| IBIS file was generated by Viper version: 2024.10.21
[IBIS Ver]   4.2
[Comment Char]   |_char
[File Name]   mcxl20_184mapbga_9x9_l25x.ibs
[File Rev]   1.0
[Date]   Thu Oct 24 12:27:40 2024
[Source]   NXP Viper 2024.10.21
[Notes]
[Disclaimer] IMPORTANT NOTICE
  This information is provided on an AS IS basis and without warranty.
  IN NO EVENT SHALL NXP BE LIABLE FOR INCIDENTAL OR CONSEQUENTIAL
  DAMAGES ARISING FROM USE OF THIS INFORMATION. THIS DISCLAIMER OF
  WARRANTY EXTENDS TO THE USER OF THE INFORMATION, AND TO THEIR CUSTOMERS
  OR USERS OF PRODUCTS  AND IS IN LIEU OF ALL WARRANTIES WHETHER EXPRESS,
  IMPLIED, OR STATUTORY, INCLUDING IMPLIED WARRANTIES OF MERCHANTABILITY
  OR FITNESS FOR PARTICULAR PURPOSE.
  NXP does not represent or warrant that the information furnished
  hereunder is free of infringement of any third party patents,
  copyrights, trade secrets, or other intellectual property rights.
  NXP does not represent or warrant that the information is free of
  defect, or that it meets any particular standard, requirements or need
  of the user of the infomation or their customers.
  NXP reserves the right to change the information in this file
  without notice.
   http://www.nxp.com
[Copyright]   (C) Copyright NXP 2004 - 2024, All Rights Reserved.
|   MCXL20_184MAPBGA_9x9_L25x
[Component]   MCXL20_184MAPBGA_9x9_L25x
[Manufacturer]   NXP
[Package]
| variable   typ   min   max
R_pkg   0.15423   0.065679   0.22133
L_pkg   2.171e-09   9.268e-10   3.289e-09
C_pkg   5.439e-13   4.158e-13   9.414e-13
[Pin] signal_name   model_name   R_pin   L_pin   C_pin
A1   P1_13   a_ip_io_3v_3p3v   0.17035   3.190e-09 4.598e-13
A2   P1_12   a_ip_io_3v_3p3v   0.17872   3.289e-09 4.578e-13
A4   P1_8   a_ip_io_3v_3p3v   0.1711   2.737e-09 4.589e-13
A6   P1_5   a_ip_io_3v_3p3v   0.147   2.098e-09 5.293e-13
A8   P1_1   a_ip_io_3v_3p3v   0.16054   2.231e-09 5.120e-13
A10   P0_17   a_ip_io_3v_3p3v   0.17426   2.236e-09 5.511e-13
A12   P0_13   a_ip_io_3v_3p3v   0.18672   2.413e-09 5.370e-13
A14   P0_11   a_ip_io_3v_3p3v   0.18543   2.630e-09 6.485e-13
A16   P0_7   a_ip_io_3v_3p3v   0.20755   2.993e-09 6.875e-13
A17   P0_6   a_ip_io_3v_3p3v   0.20761   2.937e-09 6.404e-13
B1   P1_14   a_ip_io_3v_3p3v   0.19608   3.271e-09 4.663e-13
B2   P1_11   a_ip_io_3v_3p3v   0.15597   2.797e-09 4.421e-13
B3   P1_10   a_ip_io_3v_3p3v   0.15222   2.391e-09 4.507e-13
B4   P1_9   a_ip_io_3v_3p3v   0.1519   2.545e-09 4.674e-13
B6   P1_4   a_ip_io_3v_3p3v   0.13797   1.822e-09 5.117e-13
B7   P1_3   a_ip_io_3v_3p3v   0.13944   1.902e-09 5.174e-13
B8   P1_2   a_ip_io_3v_3p3v   0.15785   2.105e-09 5.004e-13
B10   P0_16   a_ip_io_3v_3p3v   0.1414   1.899e-09 5.304e-13
B11   P0_15   a_ip_io_3v_3p3v   0.15716   2.043e-09 5.124e-13
B12   P0_14   a_ip_io_3v_3p3v   0.14993   2.047e-09 5.325e-13
B14   P0_10   a_ip_io_3v_3p3v   0.19084   2.566e-09 6.231e-13
B15   P0_9   a_ip_io_3v_3p3v   0.17659   2.485e-09 6.402e-13
B16   P0_8   a_ip_io_3v_3p3v   0.20374   2.822e-09 6.714e-13
B17   P0_5   a_ip_io_3v_3p3v   0.1786   2.546e-09 6.374e-13
C3   P1_15   a_ip_io_3v_3p3v   0.1334   2.475e-09 4.406e-13
C4   P1_7   a_ip_io_3v_3p3v   0.13148   2.019e-09 4.158e-13
C5   P1_6   a_ip_io_3v_3p3v   0.12228   1.611e-09 4.344e-13
C6   VSS   GND   NA   NA   NA
C8   P1_0   a_ip_io_3v_3p3v   0.13521   1.593e-09 5.029e-13
C9   VSS   GND   NA   NA   NA
C10   VDD   POWER   NA   NA   NA
C12   VDD_ANA_LPADC   POWER   NA   NA   NA
C13   VSS   GND   NA   NA   NA
C14   P0_12   a_ip_io_3v_3p3v   0.17111   2.212e-09 5.976e-13
C15   RESET_B   NC   0.15386   2.028e-09 5.733e-13
D1   P1_18   a_ip_io_3v_3p3v   0.22133   2.968e-09 4.908e-13
D2   P1_17   a_ip_io_3v_3p3v   0.1529   2.346e-09 4.588e-13
D3   P1_16   a_ip_io_3v_3p3v   0.14234   2.267e-09 4.313e-13
D4   VDD   POWER   NA   NA   NA
D6   VSS   GND   NA   NA   NA
D7   NC   NC   NA   NA   NA
D9   VDD   POWER   NA   NA   NA
D11   VDD_ANA_LPADC   POWER   NA   NA   NA
D12   NC   NC   NA   NA   NA
D14   VSS   GND   NA   NA   NA
D15   VSS   GND   NA   NA   NA
D16   RTC_XO   NC   0.18344   2.356e-09 5.402e-13
D17   RTC_XI   NC   0.18384   2.393e-09 5.692e-13
E4   VSS   GND   NA   NA   NA
E5   VDD   POWER   NA   NA   NA
E7   NC   NC   NA   NA   NA
E8   NC   NC   NA   NA   NA
E10   VSS   GND   NA   NA   NA
E11   NC   NC   NA   NA   NA
E13   NC   NC   NA   NA   NA
E14   POR_EXT_B   NC   0.10978   1.409e-09 5.465e-13
F1   P1_20   a_ip_io_3v_3p3v   0.18086   2.509e-09 5.643e-13
F2   P1_21   a_ip_io_3v_3p3v   0.14346   2.018e-09 5.346e-13
F3   P1_19   a_ip_io_3v_3p3v   0.12864   1.985e-09 5.199e-13
F4   VSS   GND   NA   NA   NA
F6   NC   NC   NA   NA   NA
F8   NC   NC   NA   NA   NA
F10   NC   NC   NA   NA   NA
F12   NC   NC   NA   NA   NA
F14   ATESTMODE   NC   0.11304   1.279e-09 5.081e-13
F15   P0_4   a_ip_io_3v_3p3v   0.14348   1.835e-09 5.189e-13
F16   P0_2   a_ip_io_3v_3p3v   0.13975   1.819e-09 4.673e-13
F17   P0_3   a_ip_io_3v_3p3v   0.14535   2.001e-09 5.299e-13
G2   P1_22   a_ip_io_3v_3p3v   0.13527   1.813e-09 5.193e-13
G4   NC   NC   NA   NA   NA
G5   NC   NC   NA   NA   NA
G7   NC   NC   NA   NA   NA
G11   NC   NC   NA   NA   NA
G13   VSS   GND   NA   NA   NA
G14   NC   NC   NA   NA   NA
G16   P0_1   a_ip_io_3v_3p3v   0.142   1.967e-09 5.272e-13
H1   P2_1   a_ip_io_3v_3p3v   0.15528   2.115e-09 5.171e-13
H2   P2_0   a_ip_io_3v_3p3v   0.14258   1.997e-09 5.196e-13
H3   P2_2   a_ip_io_3v_3p3v   0.11824   1.636e-09 5.203e-13
H5   VSS   GND   NA   NA   NA
H6   NC   NC   NA   NA   NA
H8   VSS   GND   NA   NA   NA
H9   VSS   GND   NA   NA   NA
H10   VSS   GND   NA   NA   NA
H12   NC   NC   NA   NA   NA
H13   VDD_CORE_AON   POWER   NA   NA   NA
H15   VOUT_RTC   POWER   0.066449  9.268e-10 5.631e-13
H16   P0_0   a_ip_io_3v_3p3v   0.11817   1.686e-09 5.084e-13
H17   VOUT_SNS   POWER   0.096977  1.574e-09 6.065e-13
J3   P2_3   a_ip_io_3v_3p3v   0.1384   1.795e-09 4.931e-13
J4   VSS   GND   NA   NA   NA
J8   VSS   GND   NA   NA   NA
J10   VSS   GND   NA   NA   NA
J14   VSS   GND   NA   NA   NA
J15   VDD_CORE_AON   POWER   NA   NA   NA
K1   P2_5   a_ip_io_3v_3p3v   0.16205   2.076e-09 4.792e-13
K2   VDD   POWER   NA   NA   NA
K3   P2_4   a_ip_io_3v_3p3v   0.11659   1.536e-09 4.922e-13
K5   NC   NC   NA   NA   NA
K6   NC   NC   NA   NA   NA
K8   VSS   GND   NA   NA   NA
K9   VSS   GND   NA   NA   NA
K10   VSS   GND   NA   NA   NA
K12   NC   NC   NA   NA   NA
K13   VDD   POWER   NA   NA   NA
K15   VSS   GND   NA   NA   NA
K16   DCDC_BUCK_LX_AON   NC   0.06933   1.352e-09 7.820e-13
K17   VSS_DCDC_BUCK   GND   NA   NA   NA
L2   VSS   GND   NA   NA   NA
L4   VDD   POWER   NA   NA   NA
L5   VSS   GND   NA   NA   NA
L7   VDD_CORE_FIXED   POWER   NA   NA   NA
L11   NC   NC   NA   NA   NA
L13   NC   NC   NA   NA   NA
L14   VDD_BAT   POWER   NA   NA   NA
L16   VDD_BAT   POWER   NA   NA   NA
M1   P2_7   a_ip_io_3v_3p3v   0.14505   2.265e-09 5.355e-13
M2   P2_6   a_ip_io_3v_3p3v   0.15877   2.334e-09 5.294e-13
M3   VSS   GND   NA   NA   NA
M4   VSS   GND   NA   NA   NA
M6   NC   NC   NA   NA   NA
M8   NC   NC   NA   NA   NA
M10   VDD   POWER   NA   NA   NA
M12   NC   NC   NA   NA   NA
M14   VSS   GND   NA   NA   NA
M15   VSS   GND   NA   NA   NA
M16   DCDC_BUCK_LX_FIXED   NC   0.065679  1.036e-09 9.414e-13
M17   VSS_DCDC_BUCK   GND   NA   NA   NA
N4   P2_8   a_ip_io_3v_3p3v   0.14427   2.164e-09 5.628e-13
N5   VSS   GND   NA   NA   NA
N7   NC   NC   NA   NA   NA
N8   NC   NC   NA   NA   NA
N10   VSS   GND   NA   NA   NA
N11   NC   NC   NA   NA   NA
N13   VSS   GND   NA   NA   NA
N14   VDD   POWER   NA   NA   NA
P1   P2_9   a_ip_io_3v_3p3v   0.15939   2.256e-09 5.746e-13
P2   P2_10   a_ip_io_3v_3p3v   0.15955   2.136e-09 5.217e-13
P3   P2_11   a_ip_io_3v_3p3v   0.12991   1.777e-09 4.989e-13
P4   VDD   POWER   NA   NA   NA
P6   VSS   GND   NA   NA   NA
P7   NC   NC   NA   NA   NA
P9   VDD_ANA   POWER   NA   NA   NA
P11   VSS   GND   NA   NA   NA
P12   NC   NC   NA   NA   NA
P14   P3_15   a_ip_io_3v_3p3v   0.1417   1.812e-09 5.514e-13
P15   P3_12   a_ip_io_3v_3p3v   0.13965   1.919e-09 5.073e-13
P16   P3_13   a_ip_io_3v_3p3v   0.15542   2.050e-09 5.457e-13
P17   P3_14   a_ip_io_3v_3p3v   0.16043   2.203e-09 5.670e-13
R3   P2_12   a_ip_io_3v_3p3v   0.17829   2.525e-09 5.424e-13
R4   VDD   POWER   NA   NA   NA
R5   VSS   GND   NA   NA   NA
R6   VDD_CORE_FIXED   POWER   NA   NA   NA
R8   P2_25   a_ip_io_3v_3p3v   0.13425   1.649e-09 5.066e-13
R9   VDD_ANA   POWER   NA   NA   NA
R10   VREFH   NC   0.1028   1.380e-09 5.570e-13
R12   P3_1   a_ip_io_3v_3p3v   0.135   1.746e-09 5.163e-13
R13   P3_2   a_ip_io_3v_3p3v   0.12852   1.785e-09 5.125e-13
R14   P3_3   a_ip_io_3v_3p3v   0.16046   2.284e-09 4.923e-13
R15   P3_11   a_ip_io_3v_3p3v   0.12561   1.727e-09 4.876e-13
T1   P2_13   a_ip_io_3v_3p3v   0.16973   2.448e-09 5.851e-13
T2   P2_16   a_ip_io_3v_3p3v   0.15512   2.189e-09 5.473e-13
T3   P2_17   a_ip_io_3v_3p3v   0.16722   2.231e-09 5.754e-13
T4   P2_18   a_ip_io_3v_3p3v   0.16507   2.238e-09 5.661e-13
T6   P2_21   a_ip_io_3v_3p3v   0.15387   1.991e-09 5.394e-13
T7   P2_22   a_ip_io_3v_3p3v   0.12306   1.660e-09 4.942e-13
T8   P2_23   a_ip_io_3v_3p3v   0.15624   2.049e-09 5.163e-13
T10   VSS   GND   NA   NA   NA
T11   VDD   POWER   NA   NA   NA
T12   P2_26   a_ip_io_3v_3p3v   0.16047   1.979e-09 5.293e-13
T14   P3_5   a_ip_io_3v_3p3v   0.16978   2.315e-09 5.209e-13
T15   P3_6   a_ip_io_3v_3p3v   0.15889   2.268e-09 5.625e-13
T16   P3_7   a_ip_io_3v_3p3v   0.18822   2.621e-09 5.655e-13
T17   P3_10   a_ip_io_3v_3p3v   0.17598   2.546e-09 5.966e-13
U1   P2_14   a_ip_io_3v_3p3v   0.20603   2.900e-09 6.439e-13
U2   P2_15   a_ip_io_3v_3p3v   0.18195   2.605e-09 6.252e-13
U4   P2_19   NC   0.20007   2.619e-09 5.795e-13
U6   P2_20   NC   0.1782   2.459e-09 5.822e-13
U8   P2_24   a_ip_io_3v_3p3v   0.15406   2.132e-09 5.320e-13
U10   VREFL   NC   0.14493   1.806e-09 5.869e-13
U12   P3_0   a_ip_io_3v_3p3v   0.16174   2.221e-09 5.456e-13
U14   P3_4   a_ip_io_3v_3p3v   0.16567   2.373e-09 5.623e-13
U16   P3_8   a_ip_io_3v_3p3v   0.20289   2.964e-09 6.656e-13
U17   P3_9   a_ip_io_3v_3p3v   0.21171   3.005e-09 6.356e-13
[Pin Mapping]   pulldown_ref   pullup_ref
A1   NC   NC
A2   NC   NC
A4   NC   NC
A6   NC   NC
A8   NC   NC
A10   NC   NC
A12   NC   NC
A14   NC   NC
A16   NC   NC
A17   NC   NC
B1   NC   NC
B2   NC   NC
B3   NC   NC
B4   NC   NC
B6   NC   NC
B7   NC   NC
B8   NC   NC
B10   NC   NC
B11   NC   NC
B12   NC   NC
B14   NC   NC
B15   NC   NC
B16   NC   NC
B17   NC   NC
C3   NC   NC
C4   NC   NC
C5   NC   NC
C6   VSS   NC
C8   NC   NC
C9   VSS   NC
C10   NC   VDD
C12   NC   VDD_ANA_LPADC
C13   VSS   NC
C14   NC   NC
C15   NC   NC
D1   NC   NC
D2   NC   NC
D3   NC   NC
D4   NC   VDD
D6   VSS   NC
D7   NC   NC
D9   NC   VDD
D11   NC   VDD_ANA_LPADC
D12   NC   NC
D14   VSS   NC
D15   VSS   NC
D16   NC   NC
D17   NC   NC
E4   VSS   NC
E5   NC   VDD
E7   NC   NC
E8   NC   NC
E10   VSS   NC
E11   NC   NC
E13   NC   NC
E14   NC   NC
F1   NC   NC
F2   NC   NC
F3   NC   NC
F4   VSS   NC
F6   NC   NC
F8   NC   NC
F10   NC   NC
F12   NC   NC
F14   NC   NC
F15   NC   NC
F16   NC   NC
F17   NC   NC
G2   NC   NC
G4   NC   NC
G5   NC   NC
G7   NC   NC
G11   NC   NC
G13   VSS   NC
G14   NC   NC
G16   NC   NC
H1   NC   NC
H2   NC   NC
H3   NC   NC
H5   VSS   NC
H6   NC   NC
H8   VSS   NC
H9   VSS   NC
H10   VSS   NC
H12   NC   NC
H13   NC   VDD_CORE_AON
H15   NC   VOUT_RTC
H16   NC   NC
H17   NC   VOUT_SNS
J3   NC   NC
J4   VSS   NC
J8   VSS   NC
J10   VSS   NC
J14   VSS   NC
J15   NC   VDD_CORE_AON
K1   NC   NC
K2   NC   VDD
K3   NC   NC
K5   NC   NC
K6   NC   NC
K8   VSS   NC
K9   VSS   NC
K10   VSS   NC
K12   NC   NC
K13   NC   VDD
K15   VSS   NC
K16   NC   NC
K17   VSS_DCDC_BUCK   NC
L2   VSS   NC
L4   NC   VDD
L5   VSS   NC
L7   NC   VDD_CORE_FIXED
L11   NC   NC
L13   NC   NC
L14   NC   VDD_BAT
L16   NC   VDD_BAT
M1   NC   NC
M2   NC   NC
M3   VSS   NC
M4   VSS   NC
M6   NC   NC
M8   NC   NC
M10   NC   VDD
M12   NC   NC
M14   VSS   NC
M15   VSS   NC
M16   NC   NC
M17   VSS_DCDC_BUCK   NC
N4   NC   NC
N5   VSS   NC
N7   NC   NC
N8   NC   NC
N10   VSS   NC
N11   NC   NC
N13   VSS   NC
N14   NC   VDD
P1   NC   NC
P2   NC   NC
P3   NC   NC
P4   NC   VDD
P6   VSS   NC
P7   NC   NC
P9   NC   VDD_ANA
P11   VSS   NC
P12   NC   NC
P14   NC   NC
P15   NC   NC
P16   NC   NC
P17   NC   NC
R3   NC   NC
R4   NC   VDD
R5   VSS   NC
R6   NC   VDD_CORE_FIXED
R8   NC   NC
R9   NC   VDD_ANA
R10   NC   NC
R12   NC   NC
R13   NC   NC
R14   NC   NC
R15   NC   NC
T1   NC   NC
T2   NC   NC
T3   NC   NC
T4   NC   NC
T6   NC   NC
T7   NC   NC
T8   NC   NC
T10   VSS   NC
T11   NC   VDD
T12   NC   NC
T14   NC   NC
T15   NC   NC
T16   NC   NC
T17   NC   NC
U1   NC   NC
U2   NC   NC
U4   NC   NC
U6   NC   NC
U8   NC   NC
U10   NC   NC
U12   NC   NC
U14   NC   NC
U16   NC   NC
U17   NC   NC
|*   Model Selector   *
[Model Selector] a_ip_io_3v_3p3v
p_io_25mhz_ds0_sr0_3p3v_mio   dse=0 sre=0 25mhz
p_io_25mhz_ds0_sr1_3p3v_mio   dse=0 sre=1 25mhz
p_io_25mhz_ds1_sr0_3p3v_mio   dse=1 sre=0 25mhz
p_io_25mhz_ds1_sr1_3p3v_mio   dse=1 sre=1 25mhz
p_io_25mhz_r40_ds0_sr0_3p3v_mio   dse=0 sre=0 25mhz_r40
p_io_25mhz_r40_ds0_sr1_3p3v_mio   dse=0 sre=1 25mhz_r40
p_io_25mhz_r40_ds1_sr0_3p3v_mio   dse=1 sre=0 25mhz_r40
p_io_25mhz_r40_ds1_sr1_3p3v_mio   dse=1 sre=1 25mhz_r40
p_io_50mhz_ds0_sr0_3p3v_mio   dse=0 sre=0 50mhz
p_io_50mhz_ds0_sr1_3p3v_mio   dse=0 sre=1 50mhz
p_io_50mhz_ds1_sr0_3p3v_mio   dse=1 sre=0 50mhz
p_io_50mhz_ds1_sr1_3p3v_mio   dse=1 sre=1 50mhz
p_io_25mhz_cap_ds0_sr0_3p3v_mio   dse=0 sre=0 25mhz_cap
p_io_25mhz_cap_ds0_sr1_3p3v_mio   dse=0 sre=1 25mhz_cap
p_io_25mhz_cap_ds1_sr0_3p3v_mio   dse=1 sre=0 25mhz_cap
p_io_25mhz_cap_ds1_sr1_3p3v_mio   dse=1 sre=1 25mhz_cap
p_io_25mhz_2mux_ds0_sr0_3p3v_mio   dse=0 sre=0 25mhz_2mux
p_io_25mhz_2mux_ds0_sr1_3p3v_mio   dse=0 sre=1 25mhz_2mux
p_io_25mhz_2mux_ds1_sr0_3p3v_mio   dse=1 sre=0 25mhz_2mux
p_io_25mhz_2mux_ds1_sr1_3p3v_mio   dse=1 sre=1 25mhz_2mux
p_io_100mhz_ds0_sr0_3p3v_mio   dse=0 sre=0 100mhz
p_io_100mhz_ds0_sr1_3p3v_mio   dse=0 sre=1 100mhz
p_io_100mhz_ds1_sr0_3p3v_mio   dse=1 sre=0 100mhz
p_io_100mhz_ds1_sr1_3p3v_mio   dse=1 sre=1 100mhz
p_io_100mhz_weftd_ds0_sr0_3p3v_mio   dse=0 sre=0 100mhz
p_io_100mhz_weftd_ds0_sr1_3p3v_mio   dse=0 sre=1 100mhz
p_io_100mhz_weftd_ds1_sr0_3p3v_mio   dse=1 sre=0 100mhz
p_io_100mhz_weftd_ds1_sr1_3p3v_mio   dse=1 sre=1 100mhz
p_io_i2c_ds00_ds10_sr0_3p3v_mio   dse0=0 dse1=0 sre=0 i2c
p_io_i2c_ds00_ds10_sr1_3p3v_mio   dse0=0 dse1=0 sre=1 i2c
p_io_i2c_ds00_ds11_sr0_3p3v_mio   dse0=0 dse1=1 sre=0 i2c
p_io_i2c_ds00_ds11_sr1_3p3v_mio   dse0=0 dse1=1 sre=1 i2c
p_io_i2c_ds01_ds10_sr0_3p3v_mio   dse0=1 dse1=0 sre=0 i2c
p_io_i2c_ds01_ds10_sr1_3p3v_mio   dse0=1 dse1=0 sre=1 i2c
p_io_i2c_ds01_ds11_sr0_3p3v_mio   dse0=1 dse1=1 sre=0 i2c
p_io_i2c_ds01_ds11_sr1_3p3v_mio   dse0=1 dse1=1 sre=1 i2c
p_io_i2c_i2c1_3p3v_mio   ipp_i2c_lv=1 i2c
p_io_i2cfmp_ds00_ds10_sr0_3p3v_mio   dse0=0 dse1=0 sre=0 i2cfmp
p_io_i2cfmp_ds00_ds10_sr1_3p3v_mio   dse0=0 dse1=0 sre=1 i2cfmp
p_io_i2cfmp_ds00_ds11_sr0_3p3v_mio   dse0=0 dse1=1 sre=0 i2cfmp
p_io_i2cfmp_ds00_ds11_sr1_3p3v_mio   dse0=0 dse1=1 sre=1 i2cfmp
p_io_i2cfmp_ds01_ds10_sr0_3p3v_mio   dse0=1 dse1=0 sre=0 i2cfmp
p_io_i2cfmp_ds01_ds10_sr1_3p3v_mio   dse0=1 dse1=0 sre=1 i2cfmp
p_io_i2cfmp_ds01_ds11_sr0_3p3v_mio   dse0=1 dse1=1 sre=0 i2cfmp
p_io_i2cfmp_ds01_ds11_sr1_3p3v_mio   dse0=1 dse1=1 sre=1 i2cfmp
p_io_i2cfmp_i2c1_3p3v_mio   ipp_i2c_lv=1 i2cfmp
p_io_rst_3p3v_mio   rst
p_io_rst_rx1p8v_3p3v_mio   rst
p_io_aon_3p3v_mio   rst
| End [Component] MCXL20_184MAPBGA_9x9_L25x
| Models and submodels in the file (49): p_io_100mhz_ds0_sr0_3p3v_mio (I/O), p_io_100mhz_ds0_sr1_3p3v_mio (I/O), p_io_100mhz_ds1_sr0_3p3v_mio (I/O), p_io_100mhz_ds1_sr1_3p3v_mio (I/O), p_io_100mhz_weftd_ds0_sr0_3p3v_mio (I/O), p_io_100mhz_weftd_ds0_sr1_3p3v_mio (I/O), p_io_100mhz_weftd_ds1_sr0_3p3v_mio (I/O), p_io_100mhz_weftd_ds1_sr1_3p3v_mio (I/O), p_io_25mhz_2mux_ds0_sr0_3p3v_mio (I/O), p_io_25mhz_2mux_ds0_sr1_3p3v_mio (I/O), p_io_25mhz_2mux_ds1_sr0_3p3v_mio (I/O), p_io_25mhz_2mux_ds1_sr1_3p3v_mio (I/O), p_io_25mhz_cap_ds0_sr0_3p3v_mio (I/O), p_io_25mhz_cap_ds0_sr1_3p3v_mio (I/O), p_io_25mhz_cap_ds1_sr0_3p3v_mio (I/O), p_io_25mhz_cap_ds1_sr1_3p3v_mio (I/O), p_io_25mhz_ds0_sr0_3p3v_mio (I/O), p_io_25mhz_ds0_sr1_3p3v_mio (I/O), p_io_25mhz_ds1_sr0_3p3v_mio (I/O), p_io_25mhz_ds1_sr1_3p3v_mio (I/O), p_io_25mhz_r40_ds0_sr0_3p3v_mio (I/O), p_io_25mhz_r40_ds0_sr1_3p3v_mio (I/O), p_io_25mhz_r40_ds1_sr0_3p3v_mio (I/O), p_io_25mhz_r40_ds1_sr1_3p3v_mio (I/O), p_io_50mhz_ds0_sr0_3p3v_mio (I/O), p_io_50mhz_ds0_sr1_3p3v_mio (I/O), p_io_50mhz_ds1_sr0_3p3v_mio (I/O), p_io_50mhz_ds1_sr1_3p3v_mio (I/O), p_io_aon_3p3v_mio (I/O), p_io_i2c_ds00_ds10_sr0_3p3v_mio (I/O), p_io_i2c_ds00_ds10_sr1_3p3v_mio (I/O), p_io_i2c_ds00_ds11_sr0_3p3v_mio (I/O), p_io_i2c_ds00_ds11_sr1_3p3v_mio (I/O), p_io_i2c_ds01_ds10_sr0_3p3v_mio (I/O), p_io_i2c_ds01_ds10_sr1_3p3v_mio (I/O), p_io_i2c_ds01_ds11_sr0_3p3v_mio (I/O), p_io_i2c_ds01_ds11_sr1_3p3v_mio (I/O), p_io_i2c_i2c1_3p3v_mio (I/O), p_io_i2cfmp_ds00_ds10_sr0_3p3v_mio (I/O), p_io_i2cfmp_ds00_ds10_sr1_3p3v_mio (I/O), p_io_i2cfmp_ds00_ds11_sr0_3p3v_mio (I/O), p_io_i2cfmp_ds00_ds11_sr1_3p3v_mio (I/O), p_io_i2cfmp_ds01_ds10_sr0_3p3v_mio (I/O), p_io_i2cfmp_ds01_ds10_sr1_3p3v_mio (I/O), p_io_i2cfmp_ds01_ds11_sr0_3p3v_mio (I/O), p_io_i2cfmp_ds01_ds11_sr1_3p3v_mio (I/O), p_io_i2cfmp_i2c1_3p3v_mio (I/O), p_io_rst_3p3v_mio (I/O), p_io_rst_rx1p8v_3p3v_mio (I/O)
